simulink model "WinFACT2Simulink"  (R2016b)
settings: Solver=ode4  StartTime=0.0  StopTime=600  FixedStep=0.01  RelTol=1e-3  EnableMultiTasking=on
libraries: instrumentlib x1

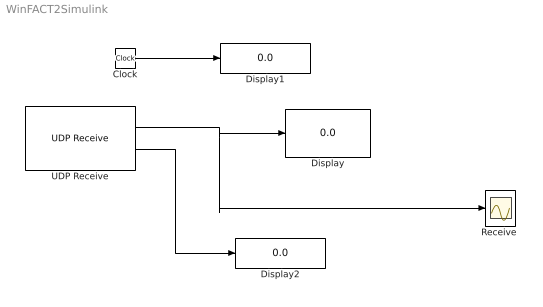
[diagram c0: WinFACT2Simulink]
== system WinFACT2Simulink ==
  Clock : Clock
  Display : Display
  Display1 : Display
  Display2 : Display
  "Receive " : Scope
  UDP Receive : instrumentlib/UDP Receive  Priority=2  Host=127.0.0.1  Port=9090  LocalPort=1600  DataSize=2  EnableBlockingMode=off  Timeout=1  SampleTime=0.01  DataType=double  ByteOrder=LittleEndian
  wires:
  Clock/1 -> Display1/1
  UDP Receive/1 -> "Receive "/1, Display/1
  UDP Receive/2 -> Display2/1
